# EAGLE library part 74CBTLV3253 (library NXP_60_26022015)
Dual 1-of-4 multiplexer/demultiplexer The 74CBTLV3253 provides a dual 1-of-4 high-speed multiplexer/demultiplexer with two common select inputs (S0, S1) and two output enable inputs (1OE, 2OE). The low ON resistance of the switch allows inputs to be connected to outputs without adding propagation delay or generating additional ground bounce noise. When pin nOE = LOW, one of the four switches is selected (low-impedance ON-state) with pins S0 and S1. When pin nOE = HIGH, all switches are in the high-impedance OFF-state, independent of pins S0 and S1. To ensure the high-impedance OFF-state during power-up or power-down, nOE should be tied to the VCC through a pull-up resistor. The minimum value of the resistor is determined by the current-sinking capability of the driver. Schmitt trigger action at control input makes the circuit tolerant to slower input rise and fall times across the entire VCC range from 2.3 V to 3.6 V. This device is fully specified for partial power-down applications using IOFF. The IOFF circuitry disables the output, preventing the damaging backflow current through the device when it is powered down. AAL Eindhoven MK
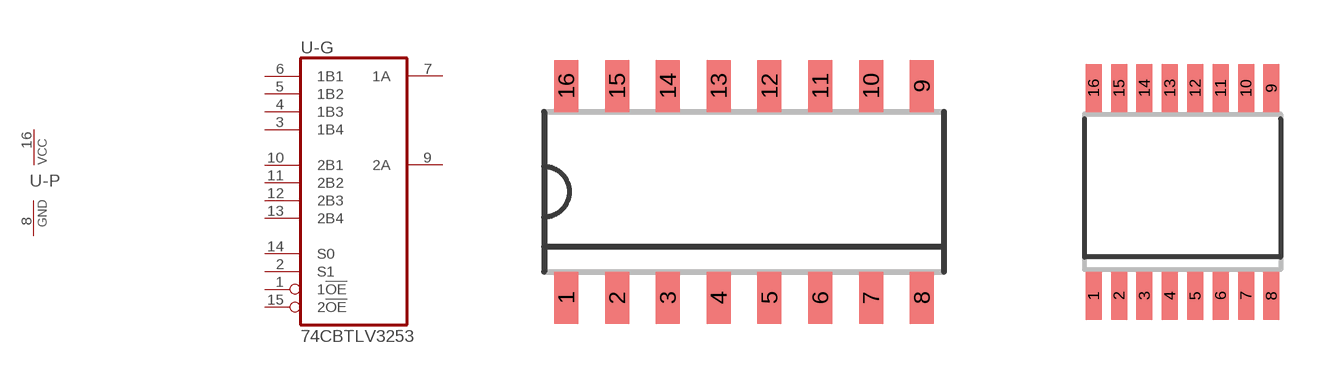
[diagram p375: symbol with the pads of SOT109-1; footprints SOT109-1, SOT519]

Designator prefix U; gates -G=74253 -P=PWRN

## 74CBTLV3253D  [SOT109-1]
1  -G:1!OE  in
2  -G:S1  in
3  -G:1B4  in
4  -G:1B3  in
5  -G:1B2  in
6  -G:1B1  in
7  -G:1A  hiz
8  -P:GND  pwr
9  -G:2A  hiz
10  -G:2B1  in
11  -G:2B2  in
12  -G:2B3  in
13  -G:2B4  in
14  -G:S0  in
15  -G:2!OE  in
16  -P:VCC  pwr

## 74CBTLV3253DS  [SOT519]
Pads as for SOT109-1

## 74CBTLV3253PW  [SOT403-1]
Pads as for SOT109-1

## 74CBTLV3253BQ  [SOT763]
1  -G:1!OE  in
2  -G:S1  in
3  -G:1B4  in
4  -G:1B3  in
5  -G:1B2  in
6  -G:1B1  in
7  -G:1A  hiz
8  -P:GND  pwr
9  -G:2A  hiz
10  -G:2B1  in
11  -G:2B2  in
12  -G:2B3  in
13  -G:2B4  in
14  -G:S0  in
15  -G:2!OE  in
16  -P:VCC  pwr
CP  -P:GND  pwr

## Footprint SOT109-1 (pad centres in mm)
SOT109-1 SO16: plastic small outline package; 16 leads; body width 3.9 mm JEDEC: MS-012 IEC: 076E07
smd 0.6 x 1.3: 1 -4.445,-2.65; 2 -3.175,-2.65; 3 -1.905,-2.65; 4 -0.635,-2.65; 5 0.635,-2.65; 6 1.905,-2.65; 7 3.175,-2.65; 8 4.445,-2.65; 9 4.445,2.65; 10 3.175,2.65; 11 1.905,2.65; 12 0.635,2.65; 13 -0.635,2.65; 14 -1.905,2.65; 15 -3.175,2.65; 16 -4.445,2.65

## Footprint SOT519 (pad centres in mm)
SOT519 SSOP16: plastic shrink small outline package; 16 leads; body width 3.9 mm; lead pitch 0.635 mm JEDEC: -- IEC: -- JEITA: --
smd 0.4 x 1.2: 1 -2.223,-2.6; 2 -1.587,-2.6; 3 -0.953,-2.6; 4 -0.318,-2.6; 5 0.318,-2.6; 6 0.953,-2.6; 7 1.587,-2.6; 8 2.223,-2.6; 9 2.223,2.6; 10 1.587,2.6; 11 0.953,2.6; 12 0.318,2.6; 13 -0.318,2.6; 14 -0.953,2.6; 15 -1.587,2.6; 16 -2.223,2.6

## Footprint SOT403-1 (pad centres in mm)
SOT403-1 TSSOP16: plastic thin shrink small outline package; 16 leads; body width 4.4 mm JEDEC: MO-153 IEC: ---
smd 0.6 x 1.35: 1 -2.375,-2.925; 8 2.375,-2.925; 9 2.375,2.925; 16 -2.375,2.925
smd 0.4 x 1.35: 2 -1.625,-2.925; 3 -0.975,-2.925; 4 -0.325,-2.925; 5 0.325,-2.925; 6 0.975,-2.925; 7 1.625,-2.925; 10 1.625,2.925; 11 0.975,2.925; 12 0.325,2.925; 13 -0.325,2.925; 14 -0.975,2.925; 15 -1.625,2.925

## Footprint SOT763 (pad centres in mm)
SOT763 DHVQFN16: plastic dual in-line compatible thermal enhanced very thin quad flat package; no leads; 16 terminals; body 2.5 x 3.5 x 0.85 mm JEDEC: MO-241 IEC: -- JEITA: --
smd 1 x 0.29: 1 -1.75,-0.25; 8 1.75,-0.25; 9 1.75,0.25; 16 -1.75,0.25
smd 0.29 x 1: 2 -1.25,-1.35; 3 -0.75,-1.35; 4 -0.25,-1.35; 5 0.25,-1.35; 6 0.75,-1.35; 7 1.25,-1.35; 10 1.25,1.35; 11 0.75,1.35; 12 0.25,1.35; 13 -0.25,1.35; 14 -0.75,1.35; 15 -1.25,1.35
smd 1.9 x 0.9: CP 0,0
